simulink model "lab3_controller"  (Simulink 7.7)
settings: Solver=VariableStepDiscrete  SolverMode=SingleTasking  StartTime=0.0  StopTime=40.0  RelTol=1e-3  AbsTol=1e-6
undefined symbols (not defined in the file or in its folder): R, T
libraries: newlab3_lib x2

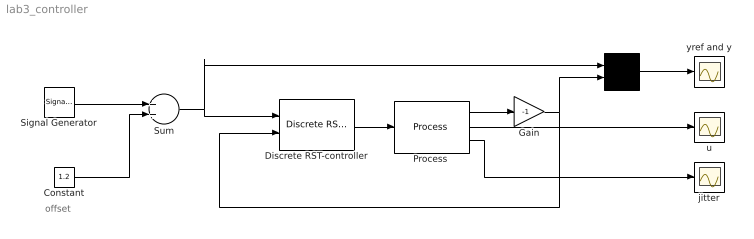
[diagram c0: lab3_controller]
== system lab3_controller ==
  note: offset
  " " : Mux  Inputs=2
  Constant : Constant  Value=1.2
  Discrete RST-controller : newlab3_lib/Discrete RST-controller  SystemSampleTime=-1  R=R  S=S  T=T  h=h
  Gain : Gain  Gain=-1
  "Process " : newlab3_lib/Process   SystemSampleTime=-1  AOu=0  AIy=0  AIu=1  h=h
  Signal Generator : SignalGenerator  WaveForm=square  Amplitude=0.1  Frequency=0.05
  Sum : Sum
  jitter : Scope
  u : Scope
  yref and y : Scope
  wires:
  Discrete RST-controller/1 -> "Process "/1
  Signal Generator/1 -> Sum/1
  Constant/1 -> Sum/2
  " "/1 -> yref and y/1
  Sum/1 -> Discrete RST-controller/1, " "/1
  "Process "/2 -> u/1
  "Process "/3 -> jitter/1
  "Process "/1 -> Gain/1
  Gain/1 -> " "/2, Discrete RST-controller/2
